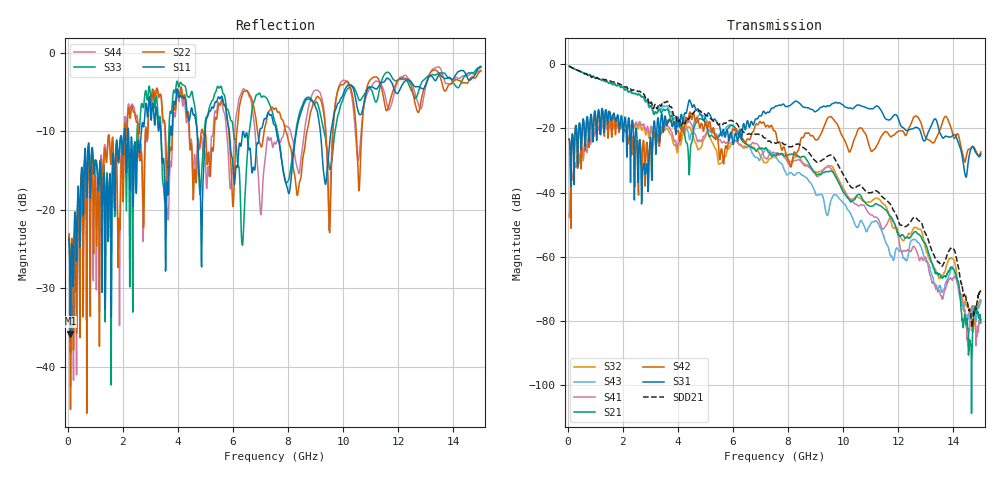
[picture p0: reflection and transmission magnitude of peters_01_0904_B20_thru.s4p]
# MHZ S RI R 50.00
! FREQ  S11  S12  S13  S14
!  S21  S22  S23  S24
!  S31  S32  S33  S34
!  S41  S42  S43  S44
!  REAL  IMAG  REAL  IMAG  REAL  IMAG  REAL  IMAG
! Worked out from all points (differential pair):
!   1496 points, 50 MHz to 15 GHz, reference 50 ohm
!   strongest paths, dB at 50 MHz, 3.79 GHz, 7.53 GHz, 11.27 GHz, 15 GHz:
!     S31: -23.3, -19.4, -13.1, -13.1, -28.0
!     S42: -23.3, -19.2, -20.8, -24.6, -27.3
!     S21: -0.6, -16.3, -28.4, -43.8, -80.7
!     S41: -47.0, -21.4, -27.7, -48.2, -79.7
!     S43: -0.6, -15.4, -28.8, -49.6, -73.9
!     S32: -47.6, -23.0, -29.0, -41.9, -73.5
!   taken as a pair (ports 1,3 in; 2,4 out), SDD21 dB: -0.5, -13.9, -24.6, -39.8, -70.6
!   lowest |S11| = -35.8 dB at 100 MHz (marker M1), VSWR 1.03, Z = 51.7 + j0.00579 ohm
!   |S11| at or under -10 dB: start of sweep to 2.054 GHz; 5.864 GHz to 6.97 GHz (1.107 GHz wide, 17.2 % of centre); 7.574 GHz to 8.307 GHz (733.8 MHz wide, 9.24 % of centre)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
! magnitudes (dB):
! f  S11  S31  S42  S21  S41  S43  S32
! 50 MHz  -23.7  -23.3  -23.3  -0.6  -47.0  -0.6  -47.6
! 100 MHz  -35.8  -33.6  -35.1  -0.8  -39.7  -0.8  -39.8
! 1.67 GHz  -13.8  -15.2  -15.3  -6.3  -19.9  -6.1  -19.8
! 2.74 GHz  -9.3  -31.9  -23.9  -10.0  -18.6  -10.3  -19.5
! 4.42 GHz  -8.6  -11.1  -15.0  -33.5  -17.7  -23.5  -19.5
! 9.59 GHz  -9.4  -12.3  -16.6  -33.4  -32.9  -41.8  -31.8
! 15 GHz  -1.9  -28.0  -27.3  -80.7  -79.7  -73.9  -73.5
